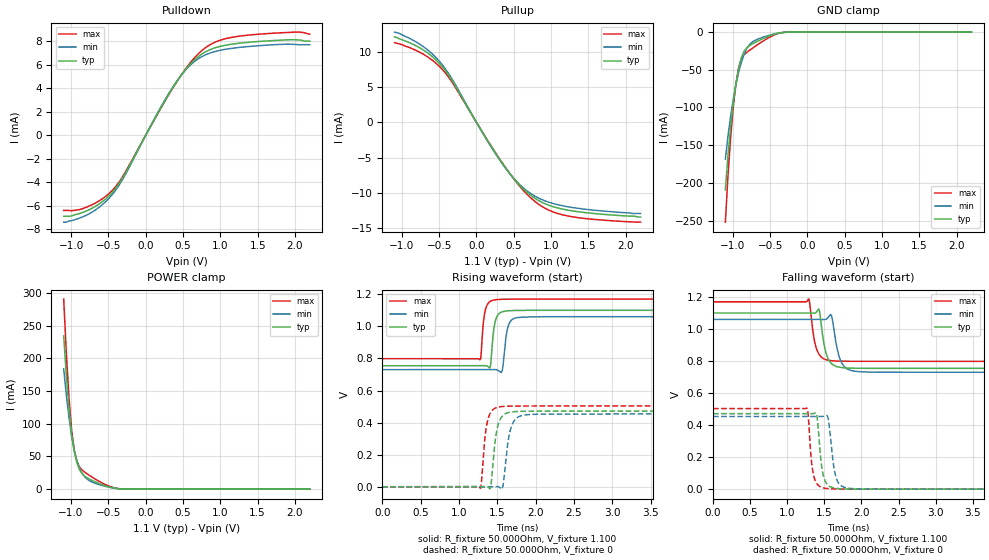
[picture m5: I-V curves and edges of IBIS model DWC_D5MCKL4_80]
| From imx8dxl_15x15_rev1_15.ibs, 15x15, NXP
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[Model] DWC_D5MCKL4_80
Model_type   I/O
Polarity   Non-Inverting
Enable   Active-High
C_comp   1.321pF   1.237pF   1.427pF
C_comp_pullup   304.579fF   285.377fF   319.196fF
C_comp_pulldown 1.005pF   946.034fF   1.122pF
Vinh = 390.000mV
Vinl = 210.000mV
Vmeas = 300.000mV
Vref = 300.000mV
Rref = 50Ohms
Cref = 0pF
[Model Spec]
Vinh   390.000mV   379.000mV   409.000mV
Vinl   210.000mV   199.000mV   229.000mV
Vmeas   300.000mV   289.000mV   319.000mV
Vref   300.000mV   289.000mV   319.000mV
D_overshoot_ampl_h 0.35 NA   NA
D_overshoot_ampl_l 0.35 NA   NA
D_overshoot_area_l 800.000p NA   NA
D_overshoot_area_h 800.000p NA   NA
[Receiver Thresholds]
Vcross_low = 205.000mV
Vcross_high = 395.000mV
Vdiff_ac = 140.000mV
Vdiff_dc = 140.000mV
Tdiffslew_ac = 10.000ns
[Temperature Range]   25.000   125.000   -40.000
[Voltage Range]   1.100V   1.060V   1.170V
[GND Clamp Reference]   0.00V   0.00V   0.00V
[C Comp Corner]
| variable   typ   min   max
C_comp 1.321pF   1.427pF   1.237pF
C_comp_pullup 304.579fF   319.196fF   285.377fF
C_comp_pulldown 1.005pF   1.122pF   946.034fF
[Pulldown Reference]   0.00V   0.00V   0.00V
[POWER Clamp Reference]   1.100V   1.060V   1.170V
[Pullup Reference]   1.100V   1.060V   1.170V
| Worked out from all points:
|   slope of the pulldown table from 0 to 0.165 V, typ, clamps not added: 86.4 ohm
|   slope of the pullup table from 0 to 0.165 V, typ, clamps not added: 57.5 ohm
|   GND clamp passes 1 mA (typ) near -0.36 V on its own axis
|   POWER clamp passes 1 mA (typ) near -0.39 V on its own axis
|   rising waveform, R_fixture 50.000Ohm, V_fixture 1.100: 20-80 % time 48.7ps typ, 54.4ps min, 45.9ps max; typ from 0.754 V to 1.1 V
|   rising waveform, R_fixture 50.000Ohm, V_fixture 0: 20-80 % time 71.6ps typ, 80.5ps min, 65ps max; typ from 0 V to 0.471 V
|   falling waveform, R_fixture 50.000Ohm, V_fixture 1.100: 20-80 % time 85.2ps typ, 95.9ps min, 79.5ps max; typ from 1.1 V to 0.754 V
|   falling waveform, R_fixture 50.000Ohm, V_fixture 0: 20-80 % time 64ps typ, 73.8ps min, 57.6ps max; typ from 0.471 V to 0 V
[GND Clamp]
-1.099V   -209.2mA   -168.4mA   -252.1mA
-1.064V   -163.4mA   -137.7mA   -190.3mA
-1.028V   -124.9mA   -111.2mA   -139.2mA
-992.7mV  -93.53mA   -88.68mA   -98.97mA
-957.3mV  -68.45mA   -69.71mA   -68.58mA
-921.8mV  -48.89mA   -53.8mA    -47.45mA
-886.4mV  -34.72mA   -40.61mA   -35.66mA
-815.5mV  -21.1mA    -22.26mA   -27.15mA
-673.6mV  -12.42mA   -9.691mA   -17.09mA
-460.9mV  -3.348mA   -2.898mA   -4.568mA
-319.1mV  -385.7uA   -561.1uA   -390.5uA
2.198V    36.46nA    642nA      5.339nA
[Power Clamp]
-1.098V   234.6mA    183.9mA    290.8mA
-1.063V   174.2mA    143.9mA    208.3mA
-1.027V   123.2mA    109.2mA    139.7mA
-991.8mV  84.12mA    80.63mA    90.23mA
-956.4mV  57.38mA    58.87mA    59.68mA
-920.9mV  40.3mA     43.02mA    42.62mA
-885.5mV  29.76mA    31.87mA    33.77mA
-814.5mV  19.66mA    18.65mA    25.86mA
-637.3mV  9.272mA    7.463mA    12.87mA
-460mV    2.471mA    2.346mA    3.441mA
-318.2mV  227.1uA    402.8uA    250.8uA
2.199V    -18.43nA   -638.2nA   -2.113nA
[Pulldown]
-1.099V   -6.9mA     -7.4mA     -6.4mA
-886.4mV  -6.658mA   -7.05mA    -6.323mA
-709.1mV  -6.179mA   -6.505mA   -5.883mA
-425.5mV  -4.706mA   -4.866mA   -4.544mA
-283.6mV  -3.353mA   -3.477mA   -3.253mA
319.1mV   3.591mA    3.654mA    3.552mA
496.4mV   5.277mA    5.269mA    5.306mA
673.6mV   6.526mA    6.368mA    6.724mA
886.4mV   7.34mA     7.038mA    7.781mA
1.135V    7.725mA    7.372mA    8.301mA
1.95V     8.12mA     7.738mA    8.754mA
2.198V    8mA        7.7mA      8.6mA
[Pullup]
-1.098V   12.1mA     12.79mA    11.3mA
-708.2mV  10.22mA    10.69mA    9.626mA
-566.4mV  9.072mA    9.431mA    8.592mA
-424.5mV  7.435mA    7.687mA    7.106mA
-318.2mV  5.772mA    5.99mA     5.553mA
284.5mV   -4.83mA    -4.92mA    -4.772mA
497.3mV   -7.909mA   -7.898mA   -7.961mA
674.5mV   -9.874mA   -9.678mA   -10.15mA
887.3mV   -11.37mA   -10.98mA   -11.97mA
1.135V    -12.23mA   -11.76mA   -13.03mA
1.526V    -12.85mA   -12.38mA   -13.69mA
2.199V    -13.4mA    -12.9mA    -14.1mA
[Ramp]
R_load=50.000Ohm
dV/dt_r   245.130mV/60.500ps  235.168mV/68.500ps  262.470mV/56.000ps
dV/dt_f   245.100mV/75.500ps  235.168mV/86.000ps  262.470mV/69.500ps
[Rising waveform]
R_fixture=50.000Ohm
V_fixture=1.100
V_fixture_min=1.060
V_fixture_max=1.170
0s        754.3mV    729.9mV    798.4mV
1.273ns   754.3mV    729.9mV    791.5mV
1.333ns   754.8mV    729.9mV    1.076V
1.403ns   740mV      729.8mV    1.154V
1.454ns   981.2mV    730.7mV    1.164V
1.494ns   1.06V      728.4mV    1.167V
1.564ns   1.091V     723.6mV    1.169V
1.654ns   1.097V     1.017V     1.169V
1.784ns   1.099V     1.056V     1.17V
10ns      1.1V       1.06V      1.17V
[Rising waveform]
R_fixture=50.000Ohm
V_fixture=0
0s        170.7nV    5.063uV    24.44nV
1.283ns   -33.32uV   5.741uV    -9.412mV
1.333ns   263.4uV    21.19uV    279.3mV
1.373ns   429uV      -23.08uV   410.8mV
1.413ns   -3.922mV   -91.12uV   463.2mV
1.484ns   325.6mV    1.08mV     492.4mV
1.554ns   433.7mV    -15.02mV   499.7mV
1.684ns   466.1mV    376.2mV    502.8mV
1.874ns   470.7mV    448.4mV    503.5mV
10ns      471.4mV    453.8mV    503.3mV
[Falling waveform]
R_fixture=50.000Ohm
V_fixture=1.100
V_fixture_min=1.060
V_fixture_max=1.170
0s        1.1V       1.06V      1.17V
1.293ns   1.1V       1.06V      1.187V
1.363ns   1.099V     1.06V      935.2mV
1.423ns   1.126V     1.06V      846mV
1.514ns   864.3mV    1.06V      809.7mV
1.584ns   790mV      1.09V      802.6mV
1.624ns   774.2mV    1.012V     800.9mV
1.734ns   759.2mV    788.1mV    799mV
1.965ns   754.8mV    733.7mV    798.2mV
10ns      754.3mV    729.8mV    798.3mV
[Falling waveform]
R_fixture=50.000Ohm
V_fixture=0
0s        471.3mV    453.7mV    503.2mV
1.263ns   471.3mV    453.7mV    506.2mV
1.323ns   471.2mV    453.7mV    186.6mV
1.363ns   472.8mV    453.7mV    72.43mV
1.403ns   449.3mV    453.7mV    31.85mV
1.474ns   111.8mV    453.9mV    9.481mV
1.544ns   27.15mV    453.7mV    3.436mV
1.654ns   5.633mV    78.82mV    846uV
1.834ns   837.6uV    5.569mV    118.7uV
10ns      308.7nV    5.349uV    127.6nV
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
